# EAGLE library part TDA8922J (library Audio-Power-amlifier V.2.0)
2 ´ 25 W class-D power amplifier
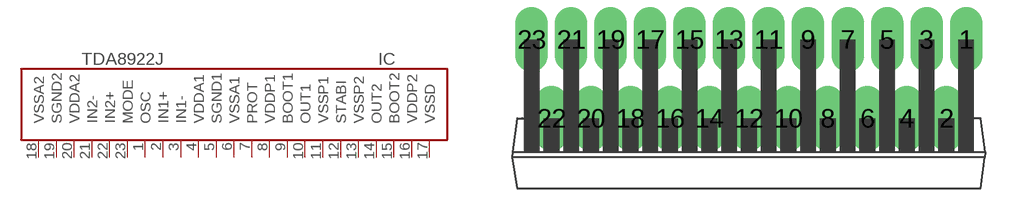
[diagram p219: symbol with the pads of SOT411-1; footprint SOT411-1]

Designator prefix IC

## TDA8922J  [SOT411-1]
1  OSC  in
2  IN1+  in
3  IN1-  in
4  VDDA1  pwr
5  SGND1  pwr
6  VSSA1  pwr
7  PROT
8  VDDP1  pwr
9  BOOT1
10  OUT1  out
11  VSSP1  pwr
12  STABI
13  VSSP2  pwr
14  OUT2  out
15  BOOT2
16  VDDP2  pwr
17  VSSD  pwr
18  VSSA2  pwr
19  SGND2  pwr
20  VDDA2  pwr
21  IN2-  in
22  IN2+  in
23  MODE  in

## Footprint SOT411-1 (pad centres in mm)
drill 1.4 long: 1 13.97,5.08; 2 12.7,0; 3 11.43,5.08; 4 10.16,0; 5 8.89,5.08; 6 7.62,0; 7 6.35,5.08; 8 5.08,0; 9 3.81,5.08; 10 2.54,0; 11 1.27,5.08; 12 0,0; 13 -1.27,5.08; 14 -2.54,0; 15 -3.81,5.08; 16 -5.08,0; 17 -6.35,5.08; 18 -7.62,0; 19 -8.89,5.08; 20 -10.16,0; 21 -11.43,5.08; 22 -12.7,0; 23 -13.97,5.08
